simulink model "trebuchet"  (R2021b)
settings: Solver=VariableStepAuto  StartTime=0.0  StopTime=3  FixedStep=0.0005  MaxStep=1e-4  RelTol=1e-4  AbsTol=1e-5  EnableMultiTasking=on
model workspace (MAT data in the model file):
  alpha0 = 0.920523020141
  finang = 45
  lsling = 20
  ppos = 6.75
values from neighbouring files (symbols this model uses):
  in = repmat(Simulink.SimulationInput(mdl),N,1)    [simulateMultipleTrebuchet.m]    (also in simulateTrebuchet.m = in.setVariable('finang',launchAngle,'workspace',mdl))
  N = 20    [simulateMultipleTrebuchet.m]
undefined symbols (not defined in the file or in its folder): deg, ft, kg, lbm, m, s, X, Y, Z
libraries: sm_lib x30, nesl_utility x5, simulink x1

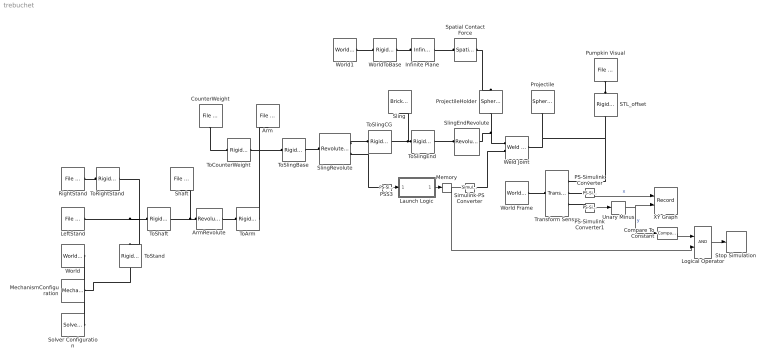
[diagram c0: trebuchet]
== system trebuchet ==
  Arm : sm_lib/Body Elements/File Solid  ExtGeomFileName=arm_prt.stl  UnitType=Custom  ExtGeomFileUnits=in  StepReaderType=HEX  ExportConvexHullGeometry=off  InertiaType=Custom  Mass=1.6  MassUnits=lbm  CenterOfMass=[2.01944889092782 0.231390262424323 -1.93537039141591e-10]  CenterOfMassUnits=in  MomentsOfInertia=[1.99947648053387 238.440492059946 240.01438453116]  MomentsOfInertiaUnits=lbm*in^2  ProductsOfInertia=[0 0 0]  ProductsOfInertiaUnits=lbm*in^2  BasedOnType=Density  Density=800  DensityUnits=kg/(m^3)  DoExposeReferenceFrame=on  SerializedFrames=<Frames/>  GraphicType=FromGeometry  MarkerShape=Sphere  MarkerSize=10  MarkerSizeUnits=m  GraphicVisPropType=SimpleVisualProperties  GraphicDiffuseColor="[0.7137    0.6078    0.2980]"  GraphicSpecularColor=[0.5 0.5 0.5 1.0]  GraphicAmbientColor=[0.15 0.15 0.15 1.0]  GraphicEmissiveColor=[0.0 0.0 0.0 1.0]  GraphicShininess=75  GraphicOpacity=1.0
  ArmRevolute : sm_lib/Joints/Revolute Joint  JointMode=Normal  SenseConstraintForce=off  SenseConstraintForceX=off  SenseConstraintForceY=off  SenseConstraintForceZ=off  SenseConstraintTorque=off  SenseConstraintTorqueX=off  SenseConstraintTorqueY=off  SenseConstraintTorqueZ=off  SenseTotalForce=off  SenseTotalForceX=off  SenseTotalForceY=off  SenseTotalForceZ=off  SenseTotalTorque=off  SenseTotalTorqueX=off  SenseTotalTorqueY=off  SenseTotalTorqueZ=off  CompositeWrenchDir=FollowerOnBase  CompositeWrenchFrame=BaseFrame  EquilibriumPosition=0  EquilibriumPositionUnits=deg  SpringStiffness=0  SpringStiffnessUnits=N*m/deg  DampingCoefficient=0  DampingCoefficientUnits=N*m/(deg/s)  TorqueActuationMode=NoTorque  MotionActuationMode=ComputedMotion  SensePosition=off  SenseVelocity=off  SenseAcceleration=off  SenseTorqueForce=off  SenseLowerLimitTorqueForce=off  SenseUpperLimitTorqueForce=off  LowerLimitSpecify=off  LowerLimitBound=-90  LowerLimitBoundUnits=deg  LowerLimitStiffness=1e4  LowerLimitStiffnessUnits=N*m/deg  LowerLimitDamping=10  LowerLimitDampingUnits=N*m/(deg/s)  LowerLimitTransitionRegionWidth=0.1  LowerLimitTransitionRegionWidthUnits=deg  UpperLimitSpecify=off  UpperLimitBound=90  UpperLimitBoundUnits=deg  UpperLimitStiffness=1e4  UpperLimitStiffnessUnits=N*m/deg  UpperLimitDamping=10  UpperLimitDampingUnits=N*m/(deg/s)  UpperLimitTransitionRegionWidth=0.1  UpperLimitTransitionRegionWidthUnits=deg  PositionTargetSpecify=on  PositionTargetPriority=High  PositionTargetValue=alpha0  PositionTargetValueUnits=rad  VelocityTargetSpecify=off  VelocityTargetPriority=High  VelocityTargetValue=0  VelocityTargetValueUnits=deg/s
  Compare To Constant : simulink/Logic and Bit Operations/Compare To Constant  relop=<=  const=-0.1  OutDataTypeStr=boolean
  CounterWeight : sm_lib/Body Elements/File Solid  ExtGeomFileName=cweight_prt.stl  UnitType=Custom  ExtGeomFileUnits=in  StepReaderType=HEX  ExportConvexHullGeometry=off  InertiaType=Custom  Mass=20  MassUnits=lbm  CenterOfMass=[0 0 0]  CenterOfMassUnits=in  MomentsOfInertia=[180.271839940582 180.271699524682 219.335621261554]  MomentsOfInertiaUnits=lbm*in^2  ProductsOfInertia=[0 0 0]  ProductsOfInertiaUnits=lbm*in^2  BasedOnType=Density  Density=8200  DensityUnits=kg/(m^3)  DoExposeReferenceFrame=on  SerializedFrames=<Frames/>  GraphicType=FromGeometry  MarkerShape=Sphere  MarkerSize=10  MarkerSizeUnits=m  GraphicVisPropType=SimpleVisualProperties  GraphicDiffuseColor=[0.5 0.5 0.5]  GraphicSpecularColor=[0.5 0.5 0.5 1.0]  GraphicAmbientColor=[0.15 0.15 0.15 1.0]  GraphicEmissiveColor=[0.0 0.0 0.0 1.0]  GraphicShininess=75  GraphicOpacity=1.0
  Infinite Plane : sm_lib/Curves and Surfaces/Infinite Plane  GraphicType=Rectangle  GraphicPlaneWidth=5  GraphicPlaneWidthUnits=m  GraphicPlaneHeight=5  GraphicPlaneHeightUnits=m  GraphicVisPropType=SimpleVisualProperties  GraphicDiffuseColor=[1 1 1]  GraphicOpacity=0.25  GraphicSpecularColor=[0.5 0.5 0.5 1.0]  GraphicAmbientColor=[0.15 0.15 0.15 1.0]  GraphicEmissiveColor=[0.0 0.0 0.0 1.0]  GraphicShininess=75
  Launch Logic : Stateflow chart  TreatAsAtomicUnit=on
  LeftStand : sm_lib/Body Elements/File Solid  ExtGeomFileName=upright_prt.stl  UnitType=Custom  ExtGeomFileUnits=in  StepReaderType=HEX  ExportConvexHullGeometry=off  InertiaType=Custom  Mass=5  MassUnits=lbm  CenterOfMass=[0 -6.3095100000000004 0.38968399999999997]  CenterOfMassUnits=in  MomentsOfInertia=[11765.6 43021.699999999997 54038.900000000001]  MomentsOfInertiaUnits=lbm*in^2  ProductsOfInertia=[1161.4200000000001 0 0]  ProductsOfInertiaUnits=lbm*in^2  BasedOnType=Density  Density=1000  DensityUnits=kg/(m^3)  DoExposeReferenceFrame=on  SerializedFrames=<Frames/>  GraphicType=FromGeometry  MarkerShape=Sphere  MarkerSize=10  MarkerSizeUnits=m  GraphicVisPropType=SimpleVisualProperties  GraphicDiffuseColor="[0.5098    0.3216    0.0039]"  GraphicSpecularColor=[0.5 0.5 0.5 1.0]  GraphicAmbientColor=[0.15 0.15 0.15 1.0]  GraphicEmissiveColor=[0.0 0.0 0.0 1.0]  GraphicShininess=75  GraphicOpacity=0.2
  Logical Operator : Logic  AllPortsSameDT=off  OutDataTypeStr=boolean
  MechanismConfiguration : sm_lib/Utilities/Mechanism Configuration  UniformGravity=Constant  GravityVector=[0 32.174 0]  GravityUnits=ft/s^2  LinearizationDelta=0.001  JointModeTransitionNonlinearIterations=2
  Memory : Memory
  PS-Simulink Converter : nesl_utility/PS-Simulink Converter  PhysicalDomain=network_engine_domain  SubClassName=ps_output  LeftPortType=input  RightPortType=output  PseudoPeriodic=off  Frequencies=[]  Unit=inherit  AffineConversion=off
  PS-Simulink Converter1 : nesl_utility/PS-Simulink Converter  PhysicalDomain=network_engine_domain  SubClassName=ps_output  LeftPortType=input  RightPortType=output  PseudoPeriodic=off  Frequencies=[]  Unit=inherit  AffineConversion=off
  PSS3 : nesl_utility/PS-Simulink Converter  PhysicalDomain=network_engine_domain  SubClassName=ps_output  LeftPortType=input  RightPortType=output  PseudoPeriodic=off  Frequencies=[]  Unit=deg  AffineConversion=off
  Projectile : sm_lib/Body Elements/Spherical Solid  GraphicAmbientColor=[0.15 0.15 0.15 1.0]  BasedOnType=Density  CenterOfMass=[0 0 0]  CenterOfMassUnits=m  GraphicDiffuseColor=[0.4 1.0 0.4]  Density=3000*10  DensityUnits=kg/m^3  DoExposeReferenceFrame=on  GraphicEmissiveColor=[0.0 0.0 0.0 1.0]  ExportEntireGeometry=off  SerializedExposedGeometries=<ExposedGeometries/>  SerializedFrames=<Frames/>  MarkerShape=Sphere  MarkerSize=10  GraphicType=FromGeometry  InertiaType=CalculateFromGeometry  Mass=0.074  MassUnits=lbm  MomentsOfInertia=[1 1 1]  MomentsOfInertiaUnits=lbm*in^2  GraphicOpacity=0.2  ProductsOfInertia=[0 0 0]  ProductsOfInertiaUnits=lbm*in^2  GraphicShininess=75  GraphicSpecularColor=[0.5 0.5 0.5 1.0]  SphereRadius=0.624  SphereRadiusUnits=in  GraphicVisPropType=SimpleVisualProperties
  ProjectileHolder : sm_lib/Body Elements/Spherical Solid  GraphicAmbientColor=[0.15 0.15 0.15 1.0]  BasedOnType=Density  CenterOfMass=[0 0 0]  CenterOfMassUnits=m  GraphicDiffuseColor=[1 0.25 0]  Density=3000  DensityUnits=kg/m^3  DoExposeReferenceFrame=on  GraphicEmissiveColor=[0.0 0.0 0.0 1.0]  ExportEntireGeometry=on  SerializedExposedGeometries=<ExposedGeometries><ExposedGeometry><RawGeometryId>entire</RawGeometryId><ExposedGeometryId>G</ExposedGeometryId></ExposedGeometry></ExposedGeometries>  SerializedFrames=<Frames/>  MarkerShape=Sphere  MarkerSize=10  GraphicType=FromGeometry  InertiaType=Custom  Mass=0.001  MassUnits=kg  MomentsOfInertia=[1 1 1]  MomentsOfInertiaUnits=lbm*in^2  GraphicOpacity=1.0  ProductsOfInertia=[0 0 0]  ProductsOfInertiaUnits=lbm*in^2  GraphicShininess=75  GraphicSpecularColor=[0.5 0.5 0.5 1.0]  SphereRadius=0.624  SphereRadiusUnits=in  GraphicVisPropType=SimpleVisualProperties
  Pumpkin Visual : sm_lib/Body Elements/File Solid  ExtGeomFileName=pumpkinskull_earring_remix.stl  UnitType=Custom  ExtGeomFileUnits=cm  StepReaderType=HEX  ExportConvexHullGeometry=off  InertiaType=PointMass  Mass=0  MassUnits=kg  CenterOfMass=[0 0 0]  CenterOfMassUnits=m  MomentsOfInertia=[1 1 1]  MomentsOfInertiaUnits=kg*m^2  ProductsOfInertia=[0 0 0]  ProductsOfInertiaUnits=kg*m^2  BasedOnType=DensityFromFile  Density=1000  DensityUnits=kg/m^3  DoExposeReferenceFrame=on  SerializedFrames=<Frames/>  GraphicType=FromGeometry  MarkerShape=Sphere  MarkerSize=10  GraphicVisPropType=SimpleVisualProperties  GraphicDiffuseColor=[1.0 0.4 0.0]  GraphicSpecularColor=[0.5 0.5 0.5 1.0]  GraphicAmbientColor=[0.15 0.15 0.15 1.0]  GraphicEmissiveColor=[0.0 0.0 0.0 1.0]  GraphicShininess=75  GraphicOpacity=1.0
  RightStand : sm_lib/Body Elements/File Solid  ExtGeomFileName=prt0002_prt.stl  UnitType=Custom  ExtGeomFileUnits=in  StepReaderType=HEX  ExportConvexHullGeometry=off  InertiaType=Custom  Mass=5  MassUnits=lbm  CenterOfMass=[0 -6.3095100000000004 -0.38968399999999997]  CenterOfMassUnits=in  MomentsOfInertia=[11765.6 43021.699999999997 54038.900000000001]  MomentsOfInertiaUnits=lbm*in^2  ProductsOfInertia=[-1161.4200000000001 0 0]  ProductsOfInertiaUnits=lbm*in^2  BasedOnType=Density  Density=1000  DensityUnits=kg/(m^3)  DoExposeReferenceFrame=on  SerializedFrames=<Frames/>  GraphicType=FromGeometry  MarkerShape=Sphere  MarkerSize=10  MarkerSizeUnits=m  GraphicVisPropType=SimpleVisualProperties  GraphicDiffuseColor="[0.5098    0.3216    0.0039]"  GraphicSpecularColor=[0.5 0.5 0.5 1.0]  GraphicAmbientColor=[0.15 0.15 0.15 1.0]  GraphicEmissiveColor=[0.0 0.0 0.0 1.0]  GraphicShininess=75  GraphicOpacity=0.2
  STL_offset : sm_lib/Frames and Transforms/Rigid Transform  TranslationMethod=Cartesian  TranslationStandardOffset=0  TranslationLengthUnit=m  TranslationStandardAxis=+Z  TranslationCartesianOffset=[-1 0 1]  TranslationROffset=0  TranslationROffsetUnits=m  TranslationZOffset=0  TranslationZOffsetUnits=m  TranslationThetaOffset=0  TranslationThetaOffsetUnits=deg  RotationMethod=StandardAxis  RotationAngleUnits=deg  RotationStandardAxis=+X  RotationAngle=-90  RotationArbitraryAxis=[0 0 1]  FollAlignAxisA=+X  BaseAlignAxisA=+Y  FollAlignAxisB=+Y  BaseAlignAxisB=+Z  RotationSequenceAxes=FollowerAxes  RotationSequence=XYX  RotationSequenceAngles=[0 0 0]  RotationSequenceAnglesUnits=deg  RotationMatrix=[1 0 0; 0 1 0; 0 0 1]
  Shaft : sm_lib/Body Elements/File Solid  ExtGeomFileName=shaft1_prt.stl  UnitType=Custom  ExtGeomFileUnits=in  StepReaderType=HEX  ExportConvexHullGeometry=off  InertiaType=Custom  Mass=0.75161  MassUnits=lbm  CenterOfMass=[0 -1.44250608133824e-19 -3.11581313569059e-16]  CenterOfMassUnits=in  MomentsOfInertia=[6.64610546204847 6.64664045415189 0.039282600271159]  MomentsOfInertiaUnits=lbm*in^2  ProductsOfInertia=[0 0 0]  ProductsOfInertiaUnits=lbm*in^2  BasedOnType=Density  Density=7850  DensityUnits=kg/(m^3)  DoExposeReferenceFrame=on  SerializedFrames=<Frames/>  GraphicType=FromGeometry  MarkerShape=Sphere  MarkerSize=10  MarkerSizeUnits=m  GraphicVisPropType=SimpleVisualProperties  GraphicDiffuseColor=[0.5 0.5 0.5]  GraphicSpecularColor=[0.5 0.5 0.5 1.0]  GraphicAmbientColor=[0.15 0.15 0.15 1.0]  GraphicEmissiveColor=[0.0 0.0 0.0 1.0]  GraphicShininess=75  GraphicOpacity=1.0
  Simulink-PS Converter : nesl_utility/Simulink-PS Converter  PhysicalDomain=network_engine_domain  SubClassName=ps_input  LeftPortType=input  RightPortType=output  PseudoPeriodic=off  Frequencies=[]  NoiseDistribution=none  NoiseParameters=[]  Unit=1  AffineConversion=off  FilteringAndDerivatives=provide  SimscapeFilterOrder=1  InputFilterTimeConstant=0.001  UdotUserProvided=0
  Sling : sm_lib/Body Elements/Brick Solid  GraphicAmbientColor=[0.15 0.15 0.15 1.0]  BasedOnType=Density  BrickDimensions=[lsling .05 .05]  BrickDimensionUnits=in  CenterOfMass=[0 0 0]  CenterOfMassUnits=m  GraphicDiffuseColor=[0.0 0 0.0]  Density=1  DensityUnits=kg/(m^3)  DoExposeReferenceFrame=on  GraphicEmissiveColor=[0.0 0.0 0.0 1.0]  ExportEntireGeometry=off  SerializedFrames=<Frames/>  MarkerShape=Sphere  MarkerSize=10  GraphicType=FromGeometry  InertiaType=CalculateFromGeometry  Mass=1  MassUnits=kg  MomentsOfInertia=[1 1 1]  MomentsOfInertiaUnits=kg*m^2  GraphicOpacity=1.0  ProductsOfInertia=[0 0 0]  ProductsOfInertiaUnits=kg*m^2  GraphicShininess=75  GraphicSpecularColor=[0.5 0.5 0.5 1.0]  GraphicVisPropType=SimpleVisualProperties
  SlingEndRevolute : sm_lib/Joints/Revolute Joint  JointMode=Normal  SenseConstraintForce=off  SenseConstraintForceX=off  SenseConstraintForceY=off  SenseConstraintForceZ=off  SenseConstraintTorque=off  SenseConstraintTorqueX=off  SenseConstraintTorqueY=off  SenseConstraintTorqueZ=off  SenseTotalForce=off  SenseTotalForceX=off  SenseTotalForceY=off  SenseTotalForceZ=off  SenseTotalTorque=off  SenseTotalTorqueX=off  SenseTotalTorqueY=off  SenseTotalTorqueZ=off  CompositeWrenchDir=FollowerOnBase  CompositeWrenchFrame=BaseFrame  EquilibriumPosition=0  EquilibriumPositionUnits=deg  SpringStiffness=0  SpringStiffnessUnits=N*m/deg  DampingCoefficient=0  DampingCoefficientUnits=N*m/(deg/s)  TorqueActuationMode=NoTorque  MotionActuationMode=ComputedMotion  SensePosition=off  SenseVelocity=off  SenseAcceleration=off  SenseTorqueForce=off  SenseLowerLimitTorqueForce=off  SenseUpperLimitTorqueForce=off  LowerLimitSpecify=off  LowerLimitBound=-90  LowerLimitBoundUnits=deg  LowerLimitStiffness=1e4  LowerLimitStiffnessUnits=N*m/deg  LowerLimitDamping=10  LowerLimitDampingUnits=N*m/(deg/s)  LowerLimitTransitionRegionWidth=0.1  LowerLimitTransitionRegionWidthUnits=deg  UpperLimitSpecify=off  UpperLimitBound=90  UpperLimitBoundUnits=deg  UpperLimitStiffness=1e4  UpperLimitStiffnessUnits=N*m/deg  UpperLimitDamping=10  UpperLimitDampingUnits=N*m/(deg/s)  UpperLimitTransitionRegionWidth=0.1  UpperLimitTransitionRegionWidthUnits=deg  PositionTargetSpecify=off  PositionTargetPriority=High  PositionTargetValue=-48.6  PositionTargetValueUnits=deg  VelocityTargetSpecify=off  VelocityTargetPriority=High  VelocityTargetValue=0  VelocityTargetValueUnits=deg/s
  SlingRevolute : sm_lib/Joints/Revolute Joint  JointMode=Normal  SenseConstraintForce=off  SenseConstraintForceX=off  SenseConstraintForceY=off  SenseConstraintForceZ=off  SenseConstraintTorque=off  SenseConstraintTorqueX=off  SenseConstraintTorqueY=off  SenseConstraintTorqueZ=off  SenseTotalForce=off  SenseTotalForceX=off  SenseTotalForceY=off  SenseTotalForceZ=off  SenseTotalTorque=off  SenseTotalTorqueX=off  SenseTotalTorqueY=off  SenseTotalTorqueZ=off  CompositeWrenchDir=FollowerOnBase  CompositeWrenchFrame=BaseFrame  EquilibriumPosition=0  EquilibriumPositionUnits=deg  SpringStiffness=0  SpringStiffnessUnits=N*m/deg  DampingCoefficient=0  DampingCoefficientUnits=N*m/(deg/s)  TorqueActuationMode=NoTorque  MotionActuationMode=ComputedMotion  SensePosition=on  SenseVelocity=off  SenseAcceleration=off  SenseTorqueForce=off  SenseLowerLimitTorqueForce=off  SenseUpperLimitTorqueForce=off  LowerLimitSpecify=off  LowerLimitBound=-90  LowerLimitBoundUnits=deg  LowerLimitStiffness=1e4  LowerLimitStiffnessUnits=N*m/deg  LowerLimitDamping=10  LowerLimitDampingUnits=N*m/(deg/s)  LowerLimitTransitionRegionWidth=0.1  LowerLimitTransitionRegionWidthUnits=deg  UpperLimitSpecify=off  UpperLimitBound=90  UpperLimitBoundUnits=deg  UpperLimitStiffness=1e4  UpperLimitStiffnessUnits=N*m/deg  UpperLimitDamping=10  UpperLimitDampingUnits=N*m/(deg/s)  UpperLimitTransitionRegionWidth=0.1  UpperLimitTransitionRegionWidthUnits=deg  PositionTargetSpecify=on  PositionTargetPriority=High  PositionTargetValue=-alpha0  PositionTargetValueUnits=rad  VelocityTargetSpecify=off  VelocityTargetPriority=High  VelocityTargetValue=0  VelocityTargetValueUnits=deg/s
  Solver Configuration : nesl_utility/Solver Configuration  PhysicalDomain=network_engine_domain  SubClassName=solver  LeftPortType=input  RightPortType=generic  Tones=[]  Harmonics=[]  SimulateNoise=off  Profile=off  UseLocalSampling=off  EnableSwitchedLinearOptims=on  FrequencyDomain=off  UseCCode=off  RelTol=0.001  AbsTol=1e-06  MinStep=1e-09  ToWorkspace=off  RevertToSquareIcSolve=off  NumHomotopyIterations=100  PhasorMode=off  PhasorModeNumHarmonics=1  DoDC=off  ResidualTolerance=1e-9  UseLocalSolver=off  LocalSolverChoice=NE_BACKWARD_EULER_ADVANCER  LocalSolverSampleTime=.001  DoFixedCost=off  MaxNonlinIter=3  MaxModeIter=2  ComputeImpulses=off  ImpulseIterations=2  LinearAlgebra=Sparse  EquationFormulation=NE_TIME_EF  DelaysMemoryBudget=1024  AutomaticFiltering=on  FilteringTimeConstant=0.001  PartitionStorageMethod=AS_NEEDED  PartitionMemoryBudget=1024  PartitionMethod=FAST
  Spatial Contact Force : sm_lib/Forces and Torques/Spatial Contact Force  CoefficientOfDynamicFriction=0.3  CoefficientOfStaticFriction=0.5  SenseContactBaseRotation=off  SenseContactBaseTranslation=off  NormalDamping=1e3  NormalDampingUnits=N/(m/s)  SenseContactFollowerRotation=off  SenseContactFollowerTranslation=off  SenseContactSignal=off  NormalStiffness=1e6  NormalStiffnessUnits=N/m  FrictionalCriticalVelocity=1e-3  FrictionalCriticalVelocityUnits=m/s  ZeroCrossDetectContactStartAndEnd=on  FrictionType=None  SenseFrictionalForceMagnitude=off  SenseNormalForceMagnitude=off  NormalForceType=SmoothSpringDamper  SenseNormalVelocity=off  SenseSeparationDistance=off  SenseTangentialVelocity=off  SenseTangentialVelocityMagnitude=off  NormalTransitionRegionWidth=1e-4  NormalTransitionRegionWidthUnits=m
  Stop Simulation : Stop
  ToArm : sm_lib/Frames and Transforms/Rigid Transform  TranslationMethod=StandardAxis  TranslationStandardOffset=ppos  TranslationLengthUnit=in  TranslationStandardAxis=+X  TranslationCartesianOffset=[16.25 0 0.5]  TranslationROffset=0  TranslationROffsetUnits=m  TranslationZOffset=0  TranslationZOffsetUnits=m  TranslationThetaOffset=0  TranslationThetaOffsetUnits=deg  RotationMethod=None  RotationAngleUnits=rad  RotationStandardAxis=+Z  RotationAngle=0  RotationArbitraryAxis=[0 0 0]  FollAlignAxisA=+X  BaseAlignAxisA=+Y  FollAlignAxisB=+Y  BaseAlignAxisB=+Z  RotationSequenceAxes=FollowerAxes  RotationSequence=XYX  RotationSequenceAngles=[0 0 0]  RotationSequenceAnglesUnits=deg  RotationMatrix=[1 0 0; 0 1 0; 0 0 1]
  ToCounterWeight : sm_lib/Frames and Transforms/Rigid Transform  TranslationMethod=Cartesian  TranslationStandardOffset=0  TranslationLengthUnit=in  TranslationStandardAxis=+Z  TranslationCartesianOffset=[0 0 0.52167589999999997]-[16.25 0 0.5]  TranslationROffset=0  TranslationROffsetUnits=m  TranslationZOffset=0  TranslationZOffsetUnits=m  TranslationThetaOffset=0  TranslationThetaOffsetUnits=deg  RotationMethod=ArbitraryAxis  RotationAngleUnits=rad  RotationStandardAxis=+Z  RotationAngle=0  RotationArbitraryAxis=[0 0 0]  FollAlignAxisA=+X  BaseAlignAxisA=+Y  FollAlignAxisB=+Y  BaseAlignAxisB=+Z  RotationSequenceAxes=FollowerAxes  RotationSequence=XYX  RotationSequenceAngles=[0 0 0]  RotationSequenceAnglesUnits=deg  RotationMatrix=[1 0 0; 0 1 0; 0 0 1]
  ToRightStand : sm_lib/Frames and Transforms/Rigid Transform  TranslationMethod=Cartesian  TranslationStandardOffset=0  TranslationLengthUnit=in  TranslationStandardAxis=+Z  TranslationCartesianOffset=[57.600000000000001 11 -9.25]-[57.600000000000001 11 -2]  TranslationROffset=0  TranslationROffsetUnits=m  TranslationZOffset=0  TranslationZOffsetUnits=m  TranslationThetaOffset=0  TranslationThetaOffsetUnits=deg  RotationMethod=None  RotationAngleUnits=deg  RotationStandardAxis=+Z  RotationAngle=0  RotationArbitraryAxis=[0 0 1]  FollAlignAxisA=+X  BaseAlignAxisA=+Y  FollAlignAxisB=+Y  BaseAlignAxisB=+Z  RotationSequenceAxes=FollowerAxes  RotationSequence=XYX  RotationSequenceAngles=[0 0 0]  RotationSequenceAnglesUnits=deg  RotationMatrix=[1 0 0; 0 1 0; 0 0 1]
  ToShaft : sm_lib/Frames and Transforms/Rigid Transform  TranslationMethod=Cartesian  TranslationStandardOffset=0  TranslationLengthUnit=in  TranslationStandardAxis=+Z  TranslationCartesianOffset=[0 9 0]-[0 0 3.625]  TranslationROffset=0  TranslationROffsetUnits=m  TranslationZOffset=0  TranslationZOffsetUnits=m  TranslationThetaOffset=0  TranslationThetaOffsetUnits=deg  RotationMethod=ArbitraryAxis  RotationAngleUnits=rad  RotationStandardAxis=+Z  RotationAngle=0  RotationArbitraryAxis=[0 0 0]  FollAlignAxisA=+X  BaseAlignAxisA=+Y  FollAlignAxisB=+Y  BaseAlignAxisB=+Z  RotationSequenceAxes=FollowerAxes  RotationSequence=XYX  RotationSequenceAngles=[0 0 0]  RotationSequenceAnglesUnits=deg  RotationMatrix=[1 0 0; 0 1 0; 0 0 1]
  ToSlingBase : sm_lib/Frames and Transforms/Rigid Transform  TranslationMethod=Cartesian  TranslationStandardOffset=0  TranslationLengthUnit=in  TranslationStandardAxis=+Z  TranslationCartesianOffset=[-17.75 0 0]  TranslationROffset=0  TranslationROffsetUnits=m  TranslationZOffset=0  TranslationZOffsetUnits=m  TranslationThetaOffset=0  TranslationThetaOffsetUnits=deg  RotationMethod=ArbitraryAxis  RotationAngleUnits=rad  RotationStandardAxis=+Z  RotationAngle=0  RotationArbitraryAxis=[0 0 0]  FollAlignAxisA=+X  BaseAlignAxisA=+Y  FollAlignAxisB=+Y  BaseAlignAxisB=+Z  RotationSequenceAxes=FollowerAxes  RotationSequence=XYX  RotationSequenceAngles=[0 0 0]  RotationSequenceAnglesUnits=deg  RotationMatrix=[1 0 0; 0 1 0; 0 0 1]
  ToSlingCG : sm_lib/Frames and Transforms/Rigid Transform  TranslationMethod=StandardAxis  TranslationStandardOffset=lsling/2  TranslationLengthUnit=in  TranslationStandardAxis=+X  TranslationCartesianOffset=[0 0 0]  TranslationROffset=0  TranslationROffsetUnits=m  TranslationZOffset=0  TranslationZOffsetUnits=m  TranslationThetaOffset=0  TranslationThetaOffsetUnits=deg  RotationMethod=None  RotationAngleUnits=deg  RotationStandardAxis=+Z  RotationAngle=0  RotationArbitraryAxis=[0 0 1]  FollAlignAxisA=+X  BaseAlignAxisA=+Y  FollAlignAxisB=+Y  BaseAlignAxisB=+Z  RotationSequenceAxes=FollowerAxes  RotationSequence=XYX  RotationSequenceAngles=[0 0 0]  RotationSequenceAnglesUnits=deg  RotationMatrix=[1 0 0; 0 1 0; 0 0 1]
  ToSlingEnd : sm_lib/Frames and Transforms/Rigid Transform  TranslationMethod=StandardAxis  TranslationStandardOffset=-lsling/2  TranslationLengthUnit=in  TranslationStandardAxis=-X  TranslationCartesianOffset=[0 0 0]  TranslationROffset=0  TranslationROffsetUnits=m  TranslationZOffset=0  TranslationZOffsetUnits=m  TranslationThetaOffset=0  TranslationThetaOffsetUnits=deg  RotationMethod=None  RotationAngleUnits=deg  RotationStandardAxis=+Z  RotationAngle=0  RotationArbitraryAxis=[0 0 1]  FollAlignAxisA=+X  BaseAlignAxisA=+Y  FollAlignAxisB=+Y  BaseAlignAxisB=+Z  RotationSequenceAxes=FollowerAxes  RotationSequence=XYX  RotationSequenceAngles=[0 0 0]  RotationSequenceAnglesUnits=deg  RotationMatrix=[1 0 0; 0 1 0; 0 0 1]
  ToStand : sm_lib/Frames and Transforms/Rigid Transform  TranslationMethod=Cartesian  TranslationStandardOffset=0  TranslationLengthUnit=in  TranslationStandardAxis=+Z  TranslationCartesianOffset=[-18 0 0]  TranslationROffset=0  TranslationROffsetUnits=m  TranslationZOffset=0  TranslationZOffsetUnits=m  TranslationThetaOffset=0  TranslationThetaOffsetUnits=deg  RotationMethod=ArbitraryAxis  RotationAngleUnits=rad  RotationStandardAxis=+Z  RotationAngle=3.1415926535897931  RotationArbitraryAxis=[1 0 0]  FollAlignAxisA=+X  BaseAlignAxisA=+Y  FollAlignAxisB=+Y  BaseAlignAxisB=+Z  RotationSequenceAxes=FollowerAxes  RotationSequence=XYX  RotationSequenceAngles=[0 0 0]  RotationSequenceAnglesUnits=deg  RotationMatrix=[1 0 0; 0 1 0; 0 0 1]
  Transform Sensor : sm_lib/Frames and Transforms/Transform Sensor  MeasurementFrame=World  SenseAngle=off  SenseAxis=off  SenseAngle1=off  SenseAngle2=off  SenseAngle3=off  SenseQ=off  SenseR=off  SenseOmegaX=off  SenseOmegaY=off  SenseOmegaZ=off  SenseOmega1=off  SenseOmega2=off  SenseOmega3=off  SenseQDot=off  SenseRDot=off  SenseAlphaX=off  SenseAlphaY=off  SenseAlphaZ=off  SenseAlpha1=off  SenseAlpha2=off  SenseAlpha3=off  SenseQDDot=off  SenseRDDot=off  SenseX=on  SenseY=on  SenseZ=off  SenseRad=off  SenseAzim=off  SenseDist=off  SenseInc=off  SenseXDot=off  SenseYDot=off  SenseZDot=off  SenseRadDot=off  SenseAzimDot=off  SenseDistDot=off  SenseIncDot=off  SenseXDDot=off  SenseYDDot=off  SenseZDDot=off  SenseRadDDot=off  SenseAzimDDot=off  SenseDistDDot=off  SenseIncDDot=off
  Unary Minus : UnaryMinus
  Weld Joint : sm_lib/Joints/Weld Joint  JointMode=ProvidedByInput  SenseConstraintForce=off  SenseConstraintForceX=off  SenseConstraintForceY=off  SenseConstraintForceZ=off  SenseConstraintTorque=off  SenseConstraintTorqueX=off  SenseConstraintTorqueY=off  SenseConstraintTorqueZ=off  SenseTotalForce=off  SenseTotalForceX=off  SenseTotalForceY=off  SenseTotalForceZ=off  SenseTotalTorque=off  SenseTotalTorqueX=off  SenseTotalTorqueY=off  SenseTotalTorqueZ=off  CompositeWrenchDir=FollowerOnBase  CompositeWrenchFrame=BaseFrame
  World : sm_lib/Frames and Transforms/World Frame
  World Frame : sm_lib/Frames and Transforms/World Frame
  World1 : sm_lib/Frames and Transforms/World Frame
  WorldToBase : sm_lib/Frames and Transforms/Rigid Transform  TranslationMethod=Cartesian  TranslationStandardOffset=0  TranslationLengthUnit=in  TranslationStandardAxis=+Z  TranslationCartesianOffset=[18 11.375 3.625]  TranslationROffset=0  TranslationROffsetUnits=m  TranslationZOffset=0  TranslationZOffsetUnits=m  TranslationThetaOffset=0  TranslationThetaOffsetUnits=deg  RotationMethod=StandardAxis  RotationAngleUnits=deg  RotationStandardAxis=+X  RotationAngle=90  RotationArbitraryAxis=[-1 0 0]  FollAlignAxisA=+X  BaseAlignAxisA=+Y  FollAlignAxisB=+Y  BaseAlignAxisB=+Z  RotationSequenceAxes=FollowerAxes  RotationSequence=XYX  RotationSequenceAngles=[0 0 0]  RotationSequenceAnglesUnits=deg  RotationMatrix=[1 0 0; 0 1 0; 0 0 1]
  XY Graph : Record  FileSettingsInternal="{\"entries\":[{\"content\":{\"excelSettings\":{\"content\":{},\"type\":\"Streamout.ExcelSettings\"}},\"type\":\"Streamout.FileSettingStorage\",\"uuid\":\"bf262f3b-21c9-456c-85fd-3be670748c37\"}],\"packageUris\":[\"http://schema.mathworks.com/mf0/streamout_blocks/R2020a\"],\"version\":\"1.0\"}"  Layout=[1 1]  SignalsInternal="{\"entries\":[{\"content\":{\"signals\":[{\"content\":{\"blockPath\":[\"trebuchet/XY Graph\"],\"channel\":[],\"dimensions\":[1],\"domain\":\"trebuchet/XY Graph\",\"lineColor\":\"#a2142f\",\"plots\":[1],\"port\":1,\"sid\":[],\"signalID\":26681,\"signalName\":\"x\"},\"type\":\"RecordBlkView.Signal\",\"uuid\":\"3189b5ce-5765-45ed-b2f1-ab2841f84834\"},{\"content\":{\"blockPath\":[\"trebuchet/XY Graph\"],\"channel\":[],\"dimensions\":[1],\"domain\":\"trebuch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"  VisualizationBindings="{\"xyplotplugin\":{\"info\":[{\"series\":[{\"bindingParametersList\":[{\"parameter\":\"X-Axis\",\"signalID\":26681,\"signalName\":\"x\"},{\"parameter\":\"Y-Axis\",\"signalID\":26684,\"signalName\":\"y\"}],\"seriesID\":50401}],\"subplotID\":1}]}}"  CompatibilityTag=XY
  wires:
  PS-Simulink Converter/1 -> XY Graph/1  "x"
  PS-Simulink Converter1/1 -> Unary Minus/1
  Unary Minus/1 -> XY Graph/2, Compare To Constant/1  "y"
  Logical Operator/1 -> Stop Simulation/1
  Compare To Constant/1 -> Logical Operator/1
  Memory/1 -> Logical Operator/2, Simulink-PS Converter/1
  Launch Logic/1(mode) -> Memory/1
  PSS3/1 -> Launch Logic/1(u)
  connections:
  ToArm/RConn1 -- ArmRevolute/RConn1
  ToSlingBase/RConn1 -- SlingRevolute/LConn1
  PSS3/LConn1 -- SlingRevolute/RConn2
  ArmRevolute/LConn1 -- ToShaft/RConn1 -- Shaft/RConn1
  MechanismConfiguration/RConn1 -- ToStand/RConn1 -- World/RConn1 -- Solver Configuration/RConn1
  ToRightStand/RConn1 -- RightStand/RConn1
  ToShaft/LConn1 -- ToRightStand/LConn1 -- LeftStand/RConn1 -- ToStand/LConn1
  ToArm/LConn1 -- Arm/RConn1 -- ToCounterWeight/RConn1 -- ToSlingBase/LConn1
  CounterWeight/RConn1 -- ToCounterWeight/LConn1
  SlingEndRevolute/LConn1 -- ToSlingEnd/RConn1
  SlingRevolute/RConn1 -- ToSlingCG/LConn1
  ToSlingEnd/LConn1 -- ToSlingCG/RConn1 -- Sling/RConn1
  ProjectileHolder/RConn1 -- SlingEndRevolute/RConn1 -- Weld Joint/LConn1
  Simulink-PS Converter/RConn1 -- Weld Joint/LConn2
  Spatial Contact Force/LConn1 -- Infinite Plane/RConn1
  Spatial Contact Force/RConn1 -- ProjectileHolder/LConn1
  WorldToBase/LConn1 -- World1/RConn1
  WorldToBase/RConn1 -- Infinite Plane/LConn1
  PS-Simulink Converter1/LConn1 -- Transform Sensor/RConn3
  Transform Sensor/RConn2 -- PS-Simulink Converter/LConn1
  World Frame/RConn1 -- Transform Sensor/LConn1
  Projectile/RConn1 -- Transform Sensor/RConn1 -- STL_offset/LConn1 -- Weld Joint/RConn1
  STL_offset/RConn1 -- Pumpkin Visual/RConn1

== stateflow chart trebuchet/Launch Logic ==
  state Engaged
    mode = 0;
  state Disengaged
    mode = -1;
  (default) -> Engaged
  Engaged -> Disengaged : [(finang + u + theta0) < 0]
  data: u input; mode output; finang parameter; theta0 constant double =122.7042
